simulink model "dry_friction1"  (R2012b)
settings: Solver=ode45  StartTime=0.0  StopTime=10.0  FixedStep=0.001  MaxStep=0.001  RelTol=1e-3
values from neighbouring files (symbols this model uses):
  f = FG    (= 500)    [coulomb_5.m]    (also in dry_friction_1.m; feder_masse_1.m = logspace(e1,e2,5000); feder_masse_11.m = logspace(e1,e2,5000); feder_masse_12.m = logspace(e1,e2,5000))
  Fu = 800    [dry_friction_1.m]
  fu = 0.02    [coulomb_1.m]    (also in coulomb_2.m; coulomb_3.m; coulomb_4.m; coulomb_5.m = 0.1)
  k = 10    [coulomb_10.m]    (also in coulomb_11.m; diff_filter_1.m = 250; diff_filter_2.m = 250; dry_friction_1.m = 2200)
  m = 400    [coulomb_1.m]    (also in coulomb_10.m = 10; coulomb_11.m = 10; coulomb_2.m; coulomb_3.m)

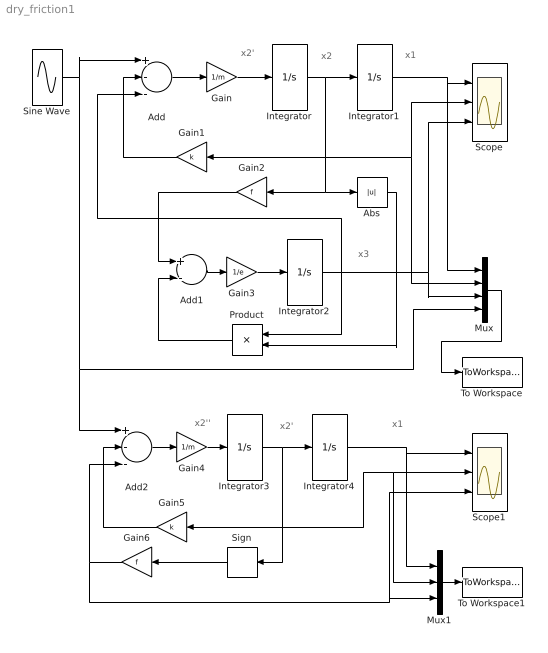
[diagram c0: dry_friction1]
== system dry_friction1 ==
  note: x1
  note: x3
  note: x1
  note: x2
  note: x2'
  note: x2'
  note: x2''
  Abs : Abs
  Add : Sum  Inputs=+--
  Add1 : Sum  Inputs=+-
  Add2 : Sum  Inputs=+--
  Gain : Gain  Gain=1/m
  Gain1 : Gain  Gain=k
  Gain2 : Gain  Gain=f
  Gain3 : Gain  Gain=1/e
  Gain4 : Gain  Gain=1/m
  Gain5 : Gain  Gain=k
  Gain6 : Gain  Gain=f
  Integrator : Integrator
  Integrator1 : Integrator
  Integrator2 : Integrator  ZeroCross=off
  Integrator3 : Integrator
  Integrator4 : Integrator  ZeroCross=off
  Mux : Mux
  Mux1 : Mux  Inputs=3
  Product : Product
  Scope : Scope  NumInputPorts=3
  Scope1 : Scope  NumInputPorts=3
  Sign : Signum  ZeroCross=off
  Sine Wave : Sin  Amplitude=Fu  Frequency=fu  SampleTime=0
  To Workspace : ToWorkspace  VariableName=y  SampleTime=-1  SaveFormat=Structure With Time
  To Workspace1 : ToWorkspace  VariableName=z  SampleTime=-1  SaveFormat=Structure With Time
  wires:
  Add/1 -> Gain/1
  Gain/1 -> Integrator/1
  Gain1/1 -> Add/2
  Gain3/1 -> Integrator2/1
  Add1/1 -> Gain3/1
  Gain2/1 -> Add1/1
  Product/1 -> Add1/2
  Abs/1 -> Product/2
  Integrator1/1 -> Mux/1, Scope/1
  Integrator/1 -> Abs/1, Gain2/1, Gain1/1, Scope/2, Mux/2, Integrator1/1
  Integrator2/1 -> Add/3, Mux/3, Scope/3, Product/1
  Mux/1 -> To Workspace/1
  Add2/1 -> Gain4/1
  Gain4/1 -> Integrator3/1
  Gain5/1 -> Add2/2
  Integrator4/1 -> Mux1/1, Scope1/1
  Integrator3/1 -> Integrator4/1, Sign/1, Gain5/1, Mux1/2, Scope1/2
  Gain6/1 -> Mux1/3, Scope1/3, Add2/3
  Mux1/1 -> To Workspace1/1
  Sine Wave/1 -> Add/1, Mux/4, Add2/1
  Sign/1 -> Gain6/1
